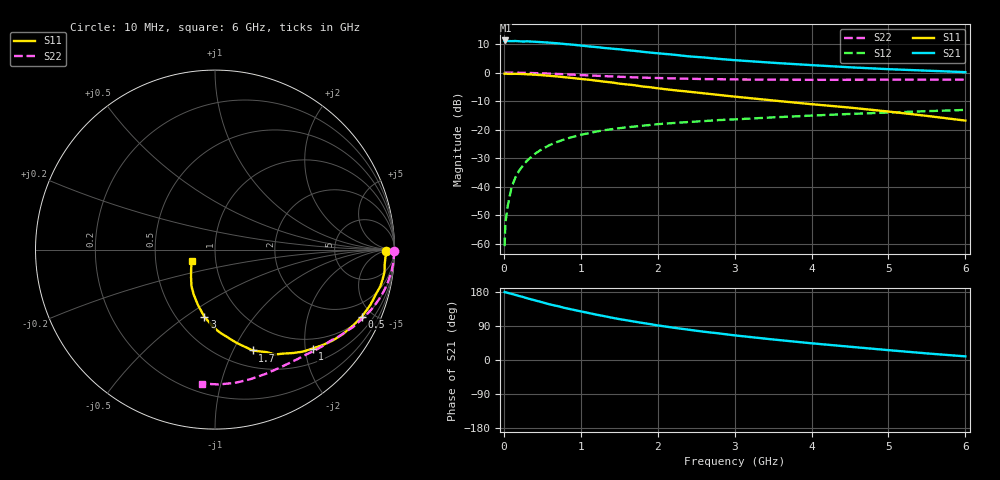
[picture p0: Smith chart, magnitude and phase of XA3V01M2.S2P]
! SIEMENS Discrete & RF Semiconductors
! BFY180
! Si NPN RF Bipolar Junction Transistor in MICRO-X
! VCE = 3 V  IC = 1.2 mA
! Common Emitter S-Parameters:  May  1997
# GHz  S  MA  R  50
!  f  S11  S21  S12  S22
! GHz  MAG  ANG  MAG  ANG  MAG  ANG  MAG  ANG
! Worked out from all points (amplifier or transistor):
!   36 points, 10 MHz to 6 GHz, reference 50 ohm
!   highest |S21| = 11.3 dB at 20 MHz (marker M1)
!   |S21| within 3 dB of that: start of sweep to 1.458 GHz
!   unconditionally stable (mu >= 1): 3.483 GHz to end of sweep
!   at 250 MHz: K = 0.09, MSG = 21.8 dB, |S12| = -32.6 dB
!   at 1.4 GHz: K = 0.54, MSG = 14.1 dB, |S12| = -19.9 dB
!   at 6 GHz: K = 1.07, MAG = 5.1 dB, |S12| = -13.1 dB
!   S11 on the Smith chart (normalised r, x): 10 MHz: 42, -8; 500 MHz: 1.11, -4.34; 1 GHz: 0.78, -2.15; 1.7 GHz: 0.68, -1.20; 3 GHz: 0.68, -0.59; 6 GHz: 0.76, -0.10
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0.01  0.9553 -0.5  3.551 179.4  0.0009 90.7  0.9976 -0.3
0.02  0.958 -1.1  3.661 178.6  0.0023 93.8  0.9999 -0.5
0.05  0.9506 -2.5  3.58 177.2  0.0045 84.3  0.9975 -1.4
0.1  0.9491 -5.0  3.558 174.6  0.0097 87.6  0.997 -2.9
0.15  0.9524 -7.6  3.579 171.8  0.0144 84.5  0.9956 -4.3
0.25  0.9441 -12.4  3.505 166.3  0.0234 82.0  0.9915 -7.0
0.3  0.9331 -14.8  3.536 163.1  0.0283 80.1  0.9874 -8.4
0.5  0.8996 -24.5  3.411 152.2  0.0457 73.5  0.969 -13.8
0.6  0.8765 -29.0  3.342 146.6  0.0538 70.4  0.9582 -16.2
0.8  0.8274 -37.9  3.163 136.9  0.0682 64.6  0.9327 -21.0
1  0.774 -45.4  2.983 128.3  0.0809 59.5  0.9045 -25.4
1.1  0.7507 -49.2  2.882 124.1  0.0861 57.1  0.8929 -27.3
1.4  0.6724 -60.3  2.632 111.8  0.1014 51.3  0.856 -32.9
1.7  0.5998 -69.5  2.406 101.2  0.113 46.5  0.8229 -37.7
2  0.5304 -77.3  2.181 91.3  0.1244 42.7  0.8035 -42.3
2.2  0.4927 -82.0  2.065 85.4  0.1301 40.2  0.7903 -45.2
2.6  0.4326 -91.1  1.842 74.6  0.1409 36.4  0.77 -50.4
3  0.3787 -99.0  1.652 65.0  0.151 33.0  0.7581 -55.5
3.5  0.3241 -106.9  1.485 54.2  0.1637 29.3  0.7498 -61.7
4.5  0.2429 -122.6  1.238 35.0  0.188 21.7  0.7483 -74.7
5.5  0.1738 -140.0  1.08 17.4  0.2104 14.2  0.7514 -88.5
6  0.1436 -154.9  1.017 9.6  0.2212 10.0  0.7499 -95.5
